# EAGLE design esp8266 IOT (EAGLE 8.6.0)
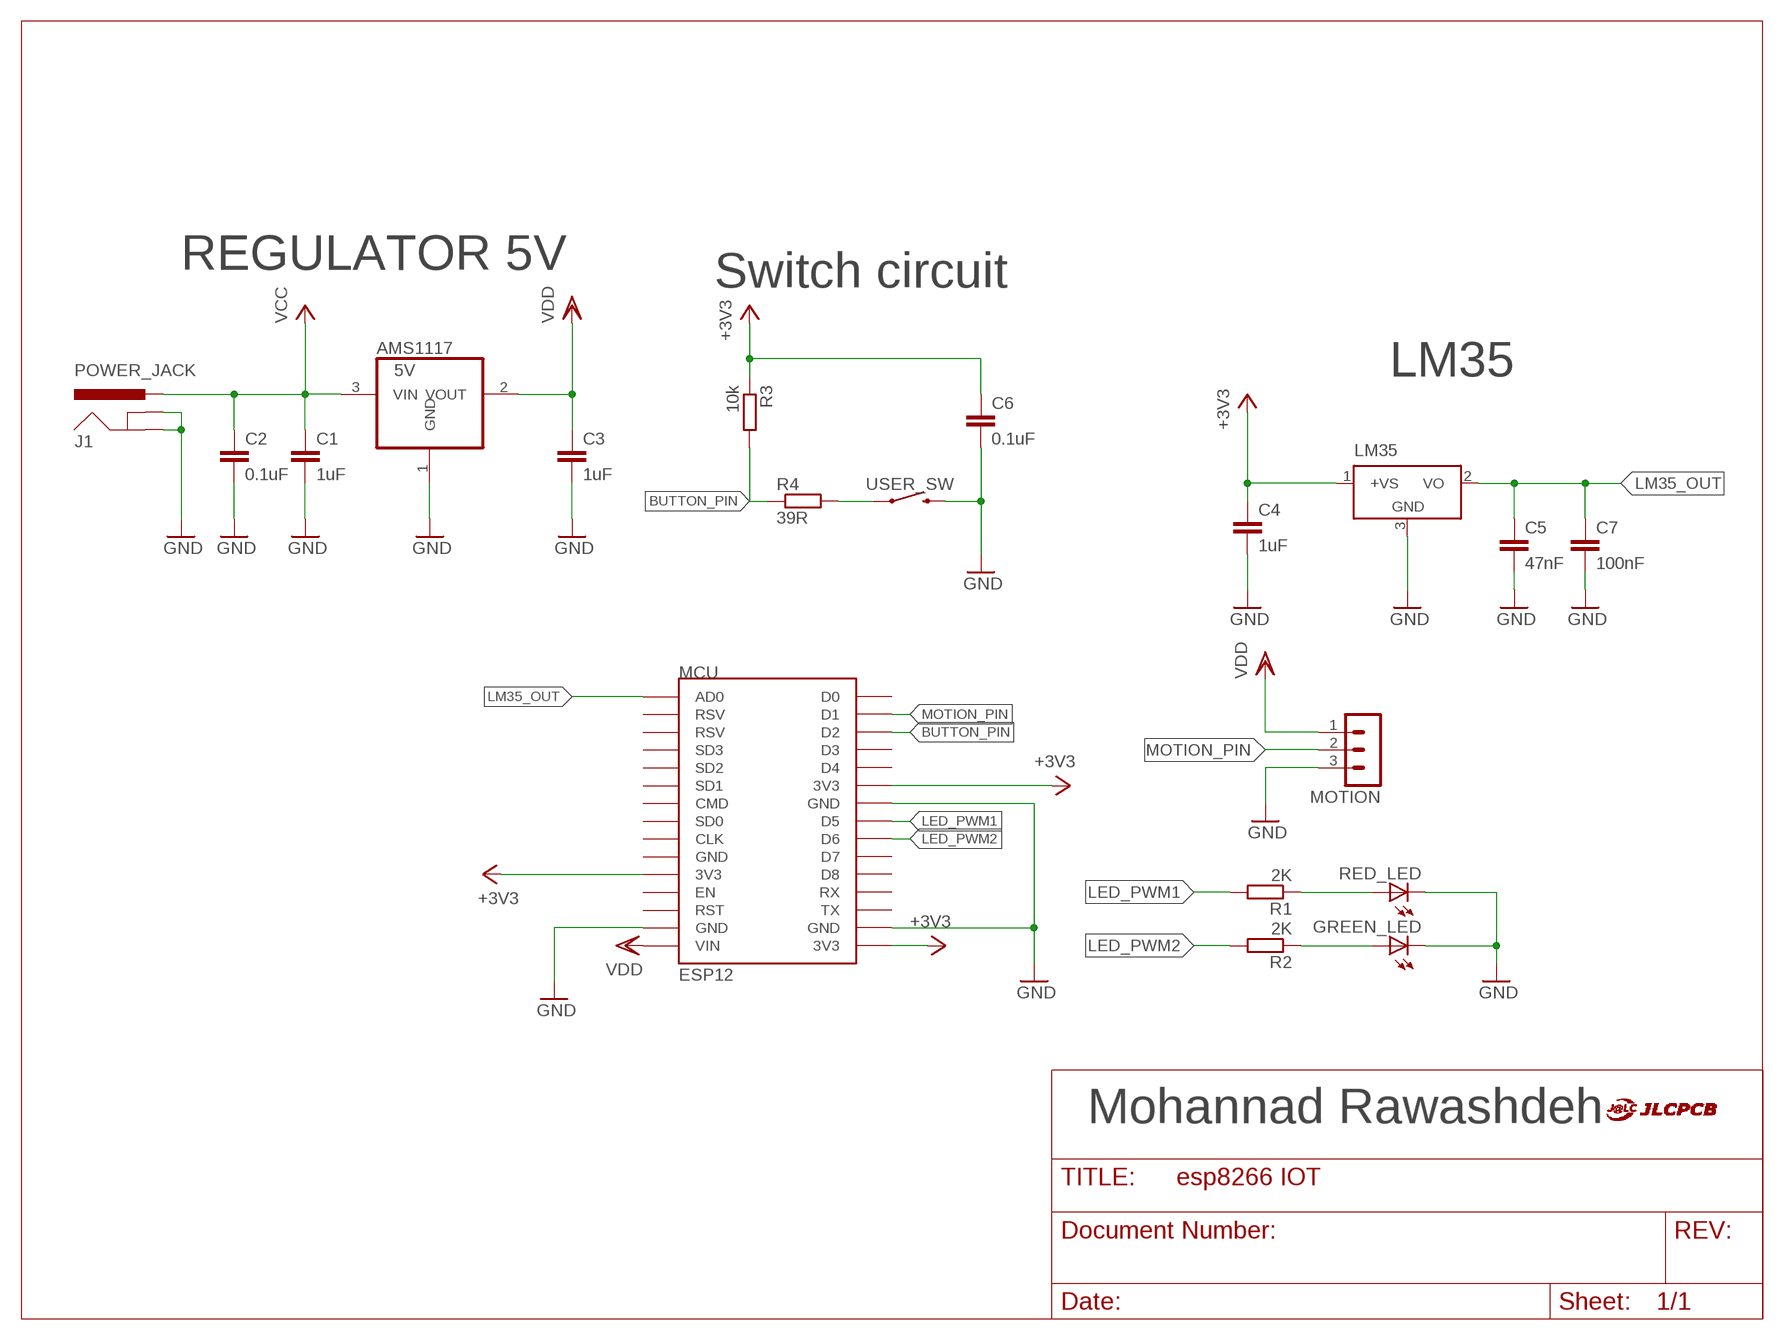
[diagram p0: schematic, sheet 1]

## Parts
AMS1117  5V  REG1117  [SOT223]
C1  1uF  C-EUC1206  [C1206]
C2  0.1uF  C-EUC1206  [C1206]
C3  1uF  C-EUC1206  [C1206]
C4  1uF  C-EUC1206  [C1206]
C5  47nF  C-EUC1206  [C1206]
C6  0.1uF  C-EUC1206  [C1206]
C7  100nF  C-EUC1206  [C1206]
GREEN_LED  LED5MM  [LED5MM]
J1  POWER_JACK  [POWER_JACK_PTH]
LM35  LM35CZ  [TO92]
MCU  ESP12  ESP12E_DEVKIT  [ESP12E_DEVKIT]
MOTION  MA03-1  [MA03-1]
R1  2K  R-EU_R1206  [R1206]
R2  2K  R-EU_R1206  [R1206]
R3  10k  R-EU_R1206  [R1206]
R4  39R  R-EU_R1206  [R1206]
RED_LED  LED5MM  [LED5MM]
U$1  JLC_LOGO  [LOGO]
USER_SW  MOMENTARY-SWITCH-SPST-SMD-5.2-REDUNDANT  [TACTILE_SWITCH_SMD_5.2MM]

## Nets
+3V3: C4.1 C6.1 LM35.1(+VS) MCU.3V3@0(3V3) MCU.3V3@1(3V3) MCU.3V3@2(3V3) R3.1
BUTTON_PIN: MCU.D2 R3.2 R4.1
GND: AMS1117.1(GND) C1.2 C2.2 C3.2 C4.2 C5.2 C6.2 C7.2 GREEN_LED.K(C) J1.GND J1.GNDBREAK LM35.3(GND) MCU.GND@1(GND) MCU.GND@2(GND) MCU.GND@3(GND) MOTION.3 RED_LED.K(C) USER_SW.3 USER_SW.4
LED_PWM1: MCU.D5 R1.2
LED_PWM2: MCU.D6 R2.2
LM35_OUT: C5.1 C7.1 LM35.2(VO) MCU.AD0
MOTION_PIN: MCU.D1 MOTION.2
N$1: GREEN_LED.A R2.1
N$3: R1.1 RED_LED.A
N$4: R4.2 USER_SW.1 USER_SW.2
VCC: AMS1117.3(VIN) C1.1 C2.1 J1.PWR
VDD: AMS1117.2(VOUT) C3.1 MCU.VIN MOTION.1
Unconnected: MCU.CLK MCU.CMD MCU.D0 MCU.D3 MCU.D4 MCU.D7 MCU.D8 MCU.EN MCU.GND@0(GND) MCU.RST MCU.RSV@0(RSV) MCU.RSV@1(RSV) MCU.RX MCU.SD0 MCU.SD1 MCU.SD2 MCU.SD3 MCU.TX

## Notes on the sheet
- REGULATOR 5V
- Switch circuit
- LM35
- Mohannad Rawashdeh

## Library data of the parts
AMS1117 = burr-brown:REG1117: 800mA and 1A Low Dropout (LDO) Positive Regulator 1.8V, 2.5V, 2.85V, 3.3V, 5V, and Adj; MPN: REG1117; OC_FARNELL: 1097566; OC_NEWARK: 14P6981
C1-C7 = rcl:C-EU: CAPACITOR, European symbol; SPICEPREFIX: C
GREEN_LED RED_LED = led:LED: LED
J1 = SparkFun-Connectors:POWER_JACK: Power Jack Connector This is the standard 5.5mm barrel jack for power. The PTH is the most common, proven, reliable, footprint. The Slot footprint only works if the mill layer is transmitted to the PCB fab house so be warned. Here are the connectors we sell at SparkFun: DC Barrel Power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; PROD_ID: CONN-08197
LM35 = lm35:LM35: Single-Supply Centigrade Temperature Sensor Vout = (10mV/°C x Temp °C) +5mmmV Source: http://www.national.com/ds/LM/LM35.pdf
MCU = ESP12E_DEVKIT:ESP12E_DEVKIT: ESP12E DEVKIT BOARD
MOTION = con-lstb:MA03-1: PIN HEADER; OC_FARNELL: unknown; OC_NEWARK: unknown
R1-R4 = rcl:R-EU_: RESISTOR, European symbol; SPICEPREFIX: R
U$1 = JLC_logo:JLC_LOGO: JLC Logo
USER_SW = SparkFun-Switches:MOMENTARY-SWITCH-SPST: Momentary Switch (Pushbutton) - SPST; PROD_ID: SWCH-08247; SF_SKU: COM-08720

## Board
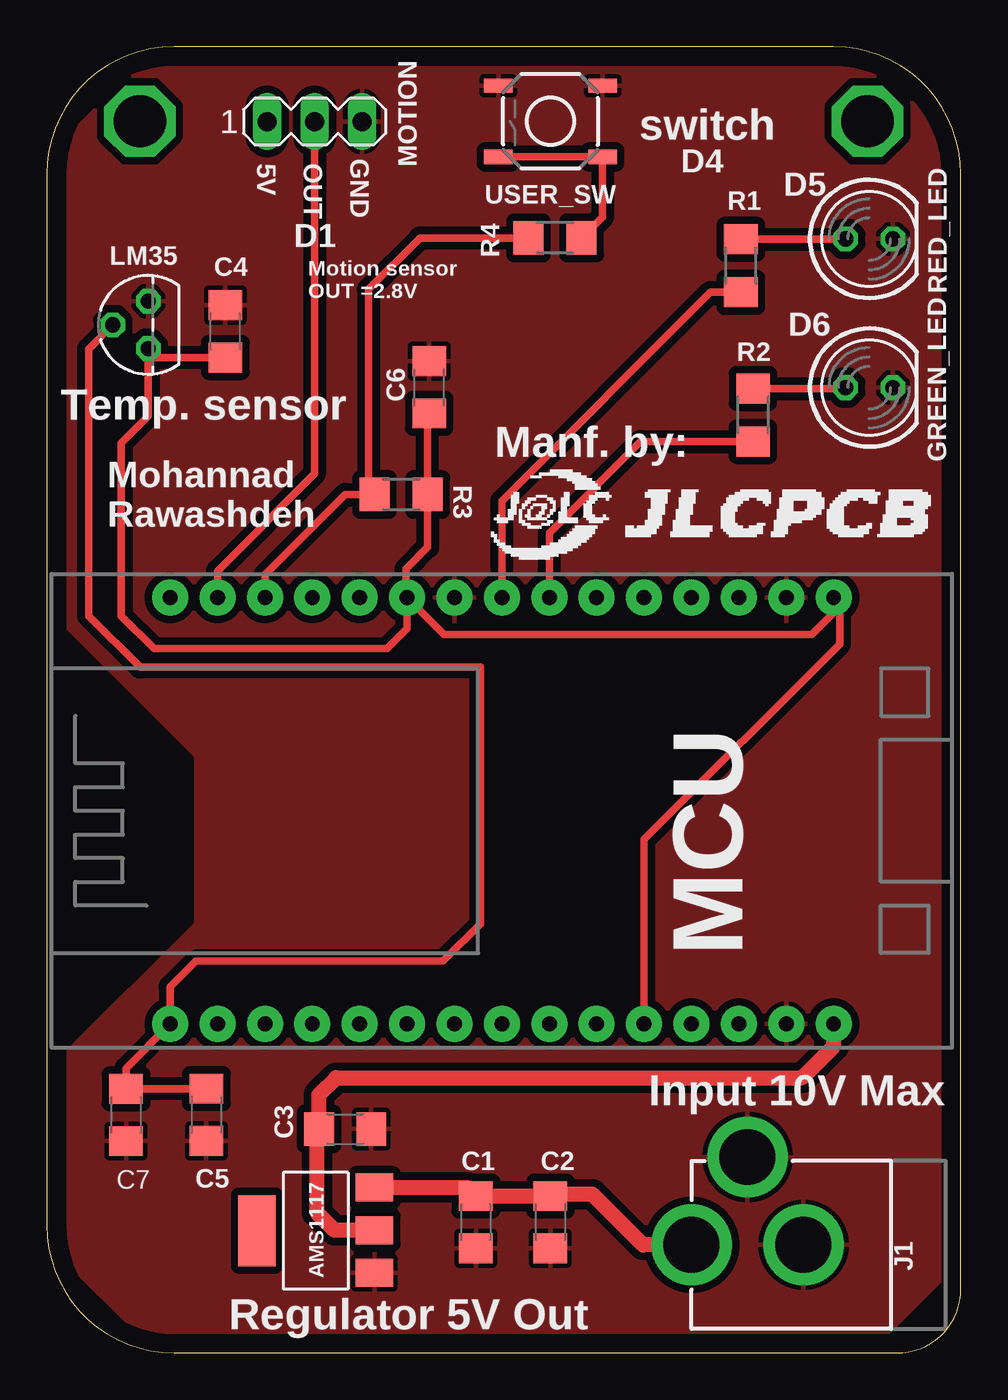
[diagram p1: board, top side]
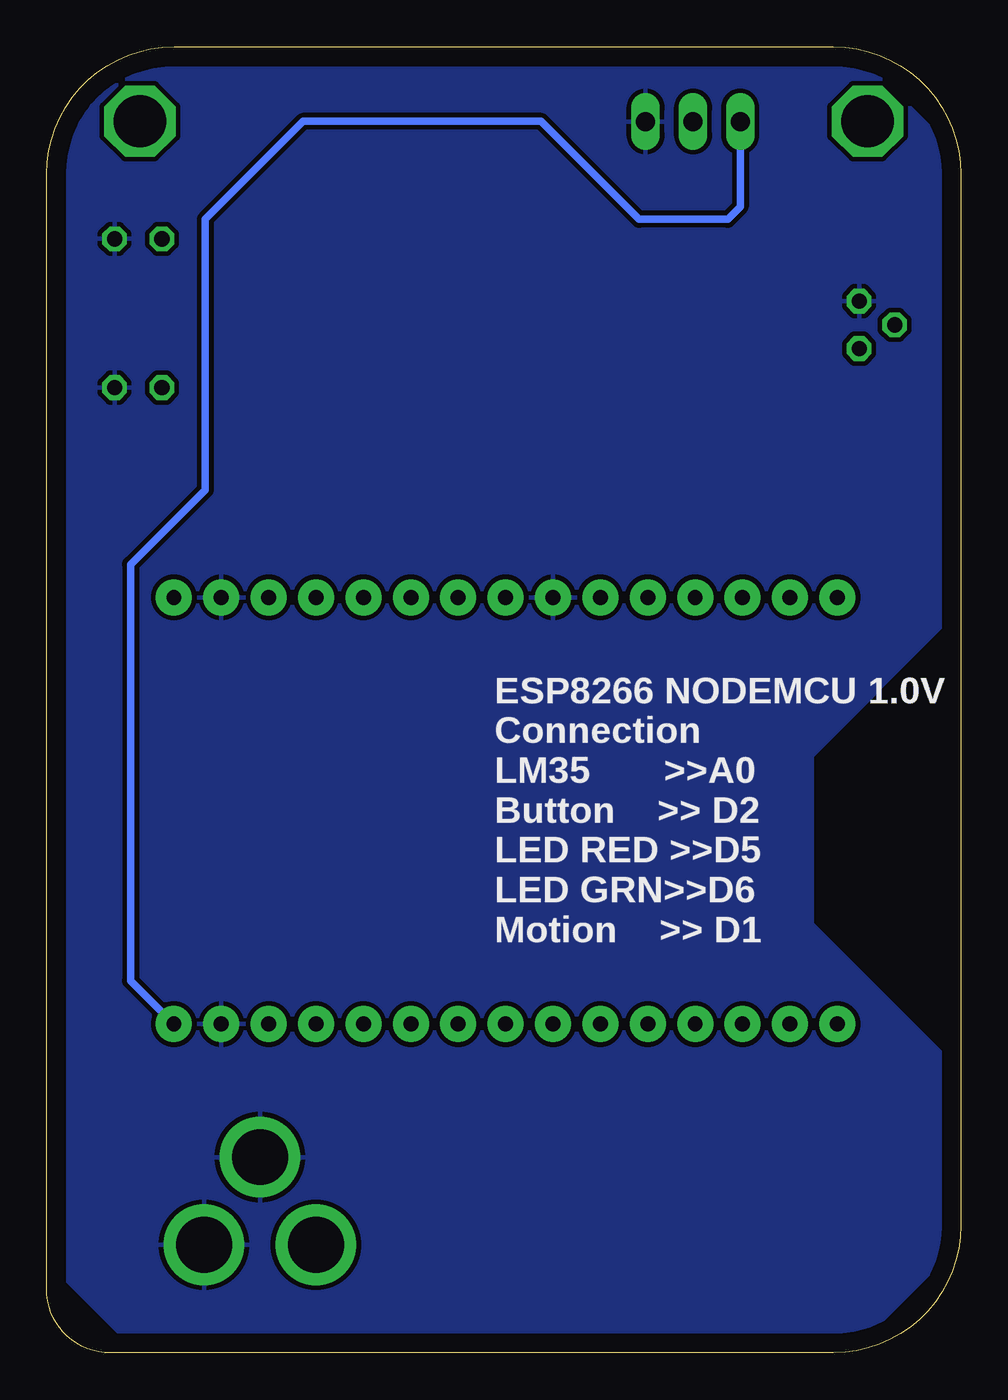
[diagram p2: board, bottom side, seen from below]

Size 49 x 70 mm. Coordinates in mm from the lower left corner, seen from the top.
Outline: 0,63.17 0,6.83 arc90 6.83,0 45.59,0 arc90 49,3.41 49,63.17 arc90 42.17,70 6.83,70 arc90 0,63.17
Copper layers (1*16): Top 0.035mm / dielectric 1.5mm / Bottom 0.035mm
Design rules "default": minimum track width 6mil, minimum drill 0.35mm, track to track 6mil, track to pad 6mil, pad to pad 6mil, via to via 6mil, smd to smd 6mil, copper to edge 40mil, drill to drill 6mil, minimum pad ring 10mil, minimum via ring 8mil, stop-mask expansion 4mil, vias tented up to drill 0mil, thermal gap 10mil

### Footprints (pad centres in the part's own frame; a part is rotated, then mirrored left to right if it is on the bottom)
SOT223 = smd 1.499 x 2.007: 1 -2.261,-3.15; 2 0.025,-3.15; 3 2.311,-3.15 | smd 3.81 x 2.007: 4 0,3.15
C1206 = smd 1.6 x 1.8: 1 -1.4,0; 2 1.4,0
LED5MM = drill 0.813 octagon: A -1.27,0; K 1.27,0
POWER_JACK_PTH = drill 2.997 pad 4.318: GND 0,7.7; GNDBREAK 4.7,10.7; PWR 0,13.7
TO92 = drill 0.813 octagon: 1 -1.27,0; 2 0,1.905; 3 1.27,0
ESP12E_DEVKIT = drill 0.8 pad 1.93: 3V3@0 -11.43,-7.62; 3V3@1 11.43,5.08; 3V3@2 11.43,-17.78; AD0 -11.43,17.78; CLK -11.43,-2.54; CMD -11.43,2.54; D0 11.43,17.78; D1 11.43,15.24; D2 11.43,12.7; D3 11.43,10.16; D4 11.43,7.62; D5 11.43,0; D6 11.43,-2.54; D7 11.43,-5.08; D8 11.43,-7.62; EN -11.43,-10.16; GND@0 -11.43,-5.08; GND@1 -11.43,-15.24; GND@2 11.43,2.54; GND@3 11.43,-15.24; RST -11.43,-12.7; RSV@0 -11.43,15.24; RSV@1 -11.43,12.7; RX 11.43,-10.16; SD0 -11.43,0; SD1 -11.43,5.08; SD2 -11.43,7.62; SD3 -11.43,10.16; TX 11.43,-12.7; VIN -11.43,-17.78
MA03-1 = drill 1.016 long: 1 -2.54,0; 2 0,0; 3 2.54,0
R1206 = smd 1.6 x 1.803: 1 -1.422,0; 2 1.422,0
TACTILE_SWITCH_SMD_5.2MM = smd 1.524 x 0.762: 1 -2.794,1.905; 2 2.794,1.905; 3 -2.794,-1.905; 4 2.794,-1.905

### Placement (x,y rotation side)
AMS1117  14.42,6.55 90 top
C1  23,7 270 top
C2  27,7 270 top
C3  16,12 0 top
C4  9.58,54.74 90 top
C5  8.56,12.76 270 top
C6  20.5,51.75 90 top
C7  4.25,12.75 270 top
GREEN_LED  44.09,51.73 0 top
J1  48.27,5.79 90 top
LM35  5.45,55.09 90 top
MCU  24.4,29.05 90 top
MOTION  14.36,65.99 0 top
R1  37.21,58.26 270 top
R2  37.86,50.26 270 top
R3  19,46 180 top
R4  27.25,59.75 0 top
RED_LED  44.09,59.7 0 top
U$1  23,42 0 top
USER_SW  27,66 180 top

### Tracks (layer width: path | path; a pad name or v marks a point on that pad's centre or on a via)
+3V3
  Top 0.406: MCU.3V3@1 19.25,40.55 19.25,42 20.42,43.17 R3.1 20.42,50.27 C6.1 | LM35.1 5.45,53.75 | 5.45,53.75 5.45,50.2 4,48.75 4,39.5 5.75,37.75 18.25,37.75 19.32,38.82 MCU.3V3@1 | C4.1 5.86,53.34 5.45,53.75 | MCU.3V3@1 21.3,38.5 41,38.5 42.18,39.68 MCU.3V3@2 42.5,40.16 42.5,38 32.02,27.52 MCU.3V3@0
BUTTON_PIN
  Top 0.406: 17.22,46 R3.2 | MCU.D2 11.7,41.7 16,46 R3.2 | R4.1 20,59.75 17.25,57 17.25,46.33 R3.2
GND
  pour Top (isolate 0.406): 5,69 45,69 48,66 48,4 45,1 5,1 1,5 1,16 8,23 8,32 1,39 1,65
  pour Bottom (isolate 0.254): 5,69 45,69 47,67 48,66 48,4 45,1 5,1 1,5 1,16 8,23 8,32 1,39 1,65
LED_PWM1
  Top 0.406: MCU.D5 24.4,45.65 35.59,56.84 R1.2
LED_PWM2
  Top 0.406: MCU.D6 26.94,43.94 31.84,48.84 R2.2
LM35_OUT
  Top 0.406: LM35.2 2.25,53.8 2.25,39.5 5,36.75 23.25,36.75 23.25,23 21.25,21 8,21 6.62,19.62 MCU.AD0 4.25,15.25 C7.1 C5.1
MOTION_PIN
  Top 0.406: MOTION.2 14.36,47.11 9.16,41.91 MCU.D1
N$1
  Top 0.406: R2.1 42.77,51.68 GREEN_LED.A
N$2  (via drill 2.8)
  other vias: 44,66
N$3
  Top 0.406: R1.1 42.8,59.68 RED_LED.A
N$4
  Top 0.406: R4.2 29.79,60.87 USER_SW.1 USER_SW.2
N$5  (via drill 2.8)
  other vias: 5,66
VCC
  Top 0.813: J1.PWR 31.96,5.79 29.25,8.5 27.1,8.5 C2.1 C1.1 22.54,8.86 AMS1117.3
VDD
  Top 0.813: AMS1117.2 15.43,6.58 14.5,7.5 14.5,11.9 C3.1 14.6,13.85 15.5,14.75 40.5,14.75 42.18,16.43 MCU.VIN
  Bottom 0.406: MOTION.1 11.82,61.43 12.5,60.75 17.25,60.75 22.5,66 35.25,66 40.5,60.75 40.5,46.25 44.5,42.25 44.5,19.94 MCU.VIN

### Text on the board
tNames: switch | 5V | OUT | GND | D4 | D5 | D1 | Motion sensor / OUT =2.8V | D6 | Temp. sensor | Manf. by: | Mohannad / Rawashdeh | Input 10V Max | Regulator 5V Out
bNames: ESP8266 NODEMCU 1.0V / Connection / LM35 >>A0 / Button >> D2 / LED RED >>D5 / LED GRN>>D6 / Motion >> D1

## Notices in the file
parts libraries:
SparkFun-Connectors: Licensing: Creative Commons ShareAlike 4.0 International - https://creativecommons.org/licenses/by-sa/4.0
